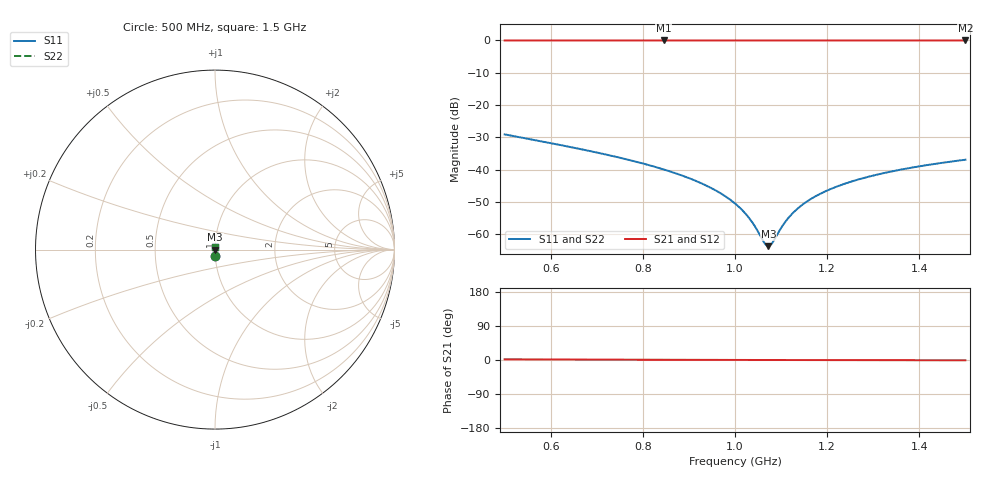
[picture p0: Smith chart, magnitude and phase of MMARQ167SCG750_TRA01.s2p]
! MMARQ167SCG750_TRA01  S-PARAMETER MODEL  ( General Type )
! Model Generated by TAIYO YUDEN Corporation (http://www.ty-top.com)
! Version 1.0
! TAIYO YUDEN Control No. 150609
! Copyright(c) 2015 TAIYO YUDEN CO.,LTD. All Rights Reserved.
! Product Description (link to TY-COMPAS)
! https://ds.yuden.co.jp/TYCOMPAS/or/detail?pn=MMARQ167SCG750JTRA01&u=M
! Products Name : Multilayer Ceramic Capacitors
! Characteristics :
!  Capacitance : 75 pF , Rated Voltage : 250V , TCC : CG / C0G
!  Case Size : 1.6 x 0.8 / 0.063 x 0.031 [mm/inch] , Thickness : 0.7 / 0.028 [mm/inch]
!  (Conditions: Temperature = 25 degC , DC Bias Current/Voltage = 0A / 0V)
! External Node Assignments :
!  1  o---| |---o  2
! GND o---------o GND
! Frequency Range : 500MHz  -  1.5GHz  [ 401 STEP ]
# MHz S RI R 50
! Freq[MHz].  S11 Real  S11 Imag  S21 Real  S21 Imag  S12 Real  S12 Imag  S22 Real  S22 Imag
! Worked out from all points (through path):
!   401 points, 500 MHz to 1.5 GHz, reference 50 ohm
!   highest |S21| = -0.01 dB at 845 MHz (marker M1); lowest = 0.0 dB at 1.5 GHz (marker M2)
!   lowest |S11| = -63.7 dB at 1.073 GHz (marker M3), VSWR 1.00, Z = 50.1 - j0.000211 ohm
!   |S11| at or under -10 dB: start of sweep to end of sweep
!   |S22| runs from -63.7 to -29.1 dB; largest |S21 - S12| = 0
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500  0.00161 -0.035  0.9984 0.035  0.9984 0.035  0.00161 -0.035
667.5  0.000864 -0.0205  0.9991 0.0205  0.9991 0.0205  0.000864 -0.0205
835  0.000633 -0.0105  0.9994 0.0105  0.9994 0.0105  0.000633 -0.0105
845  0.000627 -0.01  0.9994 0.01  0.9994 0.01  0.000627 -0.01
895  0.00061 -0.00758  0.9994 0.00758  0.9994 0.00758  0.00061 -0.00758
937.5  0.000607 -0.00562  0.9994 0.00562  0.9994 0.00562  0.000607 -0.00562
972.5  0.000611 -0.00408  0.9994 0.00408  0.9994 0.00408  0.000611 -0.00408
1000  0.000618 -0.00292  0.9994 0.00292  0.9994 0.00292  0.000618 -0.00292
1030  0.000629 -0.00168  0.9994 0.00168  0.9994 0.00168  0.000629 -0.00168
1042.5  0.000635 -0.00118  0.9994 0.00118  0.9994 0.00118  0.000635 -0.00118
1062.5  0.000645 -0.000392  0.9994 0.000392  0.9994 0.000392  0.000645 -0.000392
1067.5  0.000648 -0.000196  0.9994 0.000196  0.9994 0.000196  0.000648 -0.000196
1072.5  0.00065 -2.11e-06  0.9993 2.11e-06  0.9993 2.11e-06  0.00065 -2.11e-06
1080  0.000655 0.000288  0.9993 -0.000288  0.9993 -0.000288  0.000655 0.000288
1105  0.000671 0.00124  0.9993 -0.00124  0.9993 -0.00124  0.000671 0.00124
1122.5  0.000683 0.00189  0.9993 -0.00189  0.9993 -0.00189  0.000683 0.00189
1142.5  0.000698 0.00263  0.9993 -0.00263  0.9993 -0.00263  0.000698 0.00263
1167.5  0.000718 0.00353  0.9993 -0.00353  0.9993 -0.00353  0.000718 0.00353
1200  0.000746 0.00467  0.9993 -0.00467  0.9993 -0.00467  0.000746 0.00467
1237.5  0.000782 0.00596  0.9992 -0.00596  0.9992 -0.00596  0.000782 0.00596
1335  0.000889 0.00915  0.9991 -0.00915  0.9991 -0.00915  0.000889 0.00915
1500  0.00111 0.0142  0.9989 -0.0142  0.9989 -0.0142  0.00111 0.0142
